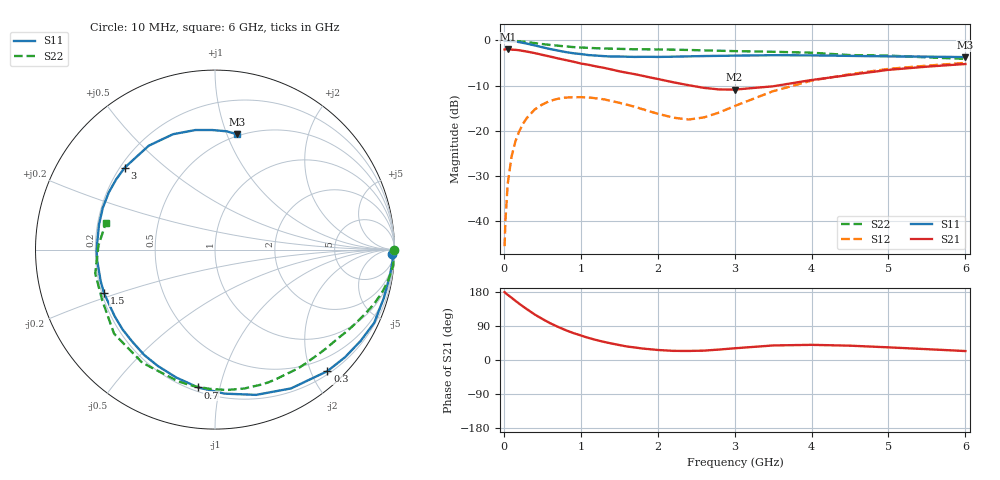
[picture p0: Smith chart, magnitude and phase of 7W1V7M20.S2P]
! Infineon Technologies  Discrete & RF Semiconductors
! BFS17W
! Si NPN RF Bipolar Junction Transistor in SOT323
! VCE = 1.75 V  IC = 0.2 mA
! Common Emitter S-Parameters:  August  1999
# GHz  S  MA  R  50
!  f  S11  S21  S12  S22
! GHz  MAG  ANG  MAG  ANG  MAG  ANG  MAG  ANG
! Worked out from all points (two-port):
!   36 points, 10 MHz to 6 GHz, reference 50 ohm
!   highest |S21| = -1.94 dB at 50 MHz (marker M1); lowest = -10.9 dB at 3 GHz (marker M2)
!   |S21| within 3 dB of the highest: start of sweep to 961.1 MHz
!   lowest |S11| = -3.7 dB at 6 GHz (marker M3), VSWR 4.78, Z = 24.3 + j54.5 ohm
!   |S11| at or under -10 dB: nowhere
!   |S22| runs from -4.1 to 0.0 dB; largest |S21 - S12| = 0.8
!   S11 on the Smith chart (normalised r, x): 10 MHz: 27, -65; 300 MHz: 0.25, -2.27; 700 MHz: 0.22, -0.86; 1.5 GHz: 0.21, -0.18; 3 GHz: 0.22, +0.37; 6 GHz: 0.49, +1.09
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0.01  0.989 -1.5  0.795 179.2  0.0053 89.0  0.9999 0.0
0.02  0.9914 -3.5  0.799 176.9  0.0099 89.6  0.9887 -0.9
0.05  0.9853 -8.1  0.8 172.0  0.0258 85.8  0.9972 -2.6
0.1  0.9785 -16.0  0.792 164.5  0.052 79.8  0.9964 -5.2
0.15  0.9764 -24.7  0.787 156.3  0.0762 73.9  0.9878 -7.8
0.3  0.9225 -47.2  0.753 134.1  0.1391 60.2  0.9595 -14.7
0.4  0.8818 -61.3  0.725 120.3  0.172 51.3  0.9355 -19.0
0.5  0.8412 -74.2  0.693 108.4  0.1957 43.6  0.9123 -22.7
0.7  0.7739 -97.0  0.634 87.8  0.2261 31.5  0.8753 -29.5
0.9  0.7225 -116.1  0.583 71.4  0.2354 21.9  0.8449 -35.8
1.1  0.689 -132.3  0.538 58.3  0.2343 14.9  0.8277 -41.9
1.5  0.6642 -158.5  0.456 39.5  0.2045 6.4  0.8077 -54.5
1.8  0.6591 -174.6  0.407 30.3  0.174 5.8  0.7982 -64.7
2.2  0.6613 167.6  0.345 24.1  0.14 17.3  0.7909 -78.2
2.6  0.6721 151.7  0.299 24.7  0.1407 40.3  0.7764 -92.2
3  0.6795 137.7  0.286 30.9  0.1882 55.1  0.7624 -105.6
3.5  0.6866 122.5  0.311 38.4  0.2746 58.0  0.7492 -122.7
4  0.6841 110.0  0.365 40.0  0.3593 52.7  0.732 -140.2
4.5  0.6751 99.3  0.416 37.8  0.4232 45.8  0.6887 -155.8
5  0.6664 91.3  0.473 33.4  0.4847 39.0  0.6804 -168.7
5.5  0.6622 84.4  0.513 28.6  0.5263 32.4  0.6496 177.9
6  0.6541 79.0  0.549 23.6  0.565 26.3  0.6258 166.3
